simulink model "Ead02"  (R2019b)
settings: Solver=FixedStepDiscrete  StartTime=0.0  StopTime=10  FixedStep=1  RelTol=1e-3

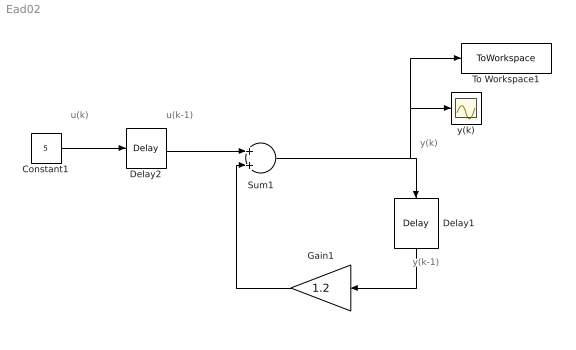
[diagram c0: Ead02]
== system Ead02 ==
  note: y(k-1)
  note: y(k)
  note: u(k)
  note: u(k-1)
  Constant1 : Constant  Value=5
  Delay1 : Delay  DelayLength=1  InitialCondition=10/1.2
  Delay2 : Delay  DelayLength=1  InitialCondition=0
  Gain1 : Gain  Gain=1.2
  Sum1 : Sum
  To Workspace1 : ToWorkspace  VariableName=y  SaveFormat=Timeseries  SampleTime=-1
  y(k) : Scope
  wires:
  Delay1/1 -> Gain1/1
  Sum1/1 -> To Workspace1/1, y(k)/1, Delay1/1
  Constant1/1 -> Delay2/1
  Gain1/1 -> Sum1/2
  Delay2/1 -> Sum1/1
